ORGANIZATION_BLOCK OB 82
TITLE = "I/O Point Fault"
AUTHOR : Esposito
FAMILY : EGAL_srl
NAME : I_0_FLT1
VERSION : 0.1


VAR_TEMP
  OB82_EV_CLASS : BYTE ;	//16#39, Event class 3, Entering event state, Internal fault event
  OB82_FLT_ID : BYTE ;	//16#XX, Fault identifcation code
  OB82_PRIORITY : BYTE ;	//26/28 (Priority of 1 is lowest)
  OB82_OB_NUMBR : BYTE ;	//82 (Organization block 82, OB82)
  OB82_RESERVED_1 : BYTE ;	//Reserved for system
  OB82_IO_FLAG : BYTE ;	//Input (01010100), Output (01010101)
  OB82_MDL_ADDR : INT ;	//Base address of module with fault
  OB82_MDL_DEFECT : BOOL ;	//Module defective
  OB82_INT_FAULT : BOOL ;	//Internal fault
  OB82_EXT_FAULT : BOOL ;	//External fault
  OB82_PNT_INFO : BOOL ;	//Point information
  OB82_EXT_VOLTAGE : BOOL ;	//External voltage low
  OB82_FLD_CONNCTR : BOOL ;	//Field wiring connector missing
  OB82_NO_CONFIG : BOOL ;	//Module has no configuration data
  OB82_CONFIG_ERR : BOOL ;	//Module has configuration error
  OB82_MDL_TYPE : BYTE ;	//Type of module
  OB82_SUB_NDL_ERR : BOOL ;	//Sub-Module is missing or has error
  OB82_COMM_FAULT : BOOL ;	//Communication fault
  OB82_MDL_STOP : BOOL ;	//Module is stopped
  OB82_WTCH_DOG_FLT : BOOL ;	//Watch dog timer stopped module
  OB82_INT_PS_FLT : BOOL ;	//Internal power supply fault
  OB82_PRIM_BATT_FLT : BOOL ;	//Primary battery is in fault
  OB82_BCKUP_BATT_FLT : BOOL ;	//Backup battery is in fault
  OB82_RESERVED_2 : BOOL ;	//Reserved for system
  OB82_RACK_FLT : BOOL ;	//Rack fault, only for bus interface module
  OB82_PROC_FLT : BOOL ;	//Processor fault
  OB82_EPROM_FLT : BOOL ;	//EPROM fault
  OB82_RAM_FLT : BOOL ;	//RAM fault
  OB82_ADU_FLT : BOOL ;	//ADU fault
  OB82_FUSE_FLT : BOOL ;	//Fuse fault
  OB82_HW_INTR_FLT : BOOL ;	//Hardware interupt input in fault
  OB82_RESERVED_3 : BOOL ;	//Reserved for system
  OB82_DATE_TIME : DATE_AND_TIME ;	//Date and time OB82 started
END_VAR
BEGIN
NETWORK
TITLE =



END_ORGANIZATION_BLOCK

